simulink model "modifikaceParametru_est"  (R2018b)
settings: Solver=ode4  StartTime=0.0  StopTime=T  FixedStep=1e-3  RelTol=1e-3
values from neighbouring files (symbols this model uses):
  b_1 = params.b_1    [mainSkript_modifikaceParametru.m]    (also in mainSkript_rovniceSystemu.m; mainSkript_overeniRovnic.m; mainSkript_kyvadlaNajednouOdhad.m; mainSkript_simulaceLQG.m)
  b_2 = params.b_2    [mainSkript_modifikaceParametru.m]    (also in mainSkript_rovniceSystemu.m; mainSkript_overeniRovnic.m; mainSkript_kyvadlaNajednouOdhad.m; mainSkript_simulaceLQG.m)
  g = 9.81    [mainSkript_modifikaceParametru.m]    (also in mainSkript_rovniceSystemu.m; mainSkript_overeniRovnic.m; mainSkript_estimaceVozik.m; mainSkript_odhadKyvadlaZvlast.m)
  I_1 = params.I_1    [mainSkript_modifikaceParametru.m]    (also in mainSkript_rovniceSystemu.m; mainSkript_overeniRovnic.m; mainSkript_kyvadlaNajednouOdhad.m; mainSkript_simulaceLQG.m)
  I_2 = params.I_2    [mainSkript_modifikaceParametru.m]    (also in mainSkript_rovniceSystemu.m; mainSkript_overeniRovnic.m; mainSkript_kyvadlaNajednouOdhad.m; mainSkript_simulaceLQG.m)
  L_1 = params.L_1    [mainSkript_modifikaceParametru.m]    (also in mainSkript_rovniceSystemu.m; mainSkript_overeniRovnic.m; odhadovane_parametry.m = 0.228; mainSkript_kyvadlaNajednouOdhad.m)
  l_1 = params.l_1    [mainSkript_modifikaceParametru.m]    (also in mainSkript_rovniceSystemu.m; mainSkript_overeniRovnic.m; odhadovane_parametry.m = 0.134; mainSkript_kyvadlaNajednouOdhad.m)
  l_2 = params.l_2    [mainSkript_modifikaceParametru.m]    (also in mainSkript_rovniceSystemu.m; mainSkript_overeniRovnic.m; odhadovane_parametry.m = 0.112; mainSkript_kyvadlaNajednouOdhad.m)
  m_1 = params.m_1    [mainSkript_modifikaceParametru.m]    (also in mainSkript_rovniceSystemu.m; mainSkript_overeniRovnic.m; mainSkript_kyvadlaNajednouOdhad.m; mainSkript_simulaceLQG.m)
  m_2 = params.m_2    [mainSkript_modifikaceParametru.m]    (also in mainSkript_rovniceSystemu.m; mainSkript_overeniRovnic.m; mainSkript_kyvadlaNajednouOdhad.m; mainSkript_simulaceLQG.m)
  q_0 = [0 pi pi 0 0 0]    [mainSkript_modifikaceParametru.m]    (also in mainSkript_kyvadlaNajednouOdhad.m = cell(1, k); mainSkript_simulaceLQG.m = [0 th1_0 th2_0 0 dth1_0 dth2_0]; mainSkript_LQGexperiment.m = zeros(6,1); mainSkript_LQGexperiment_integral.m = zeros(6,1))

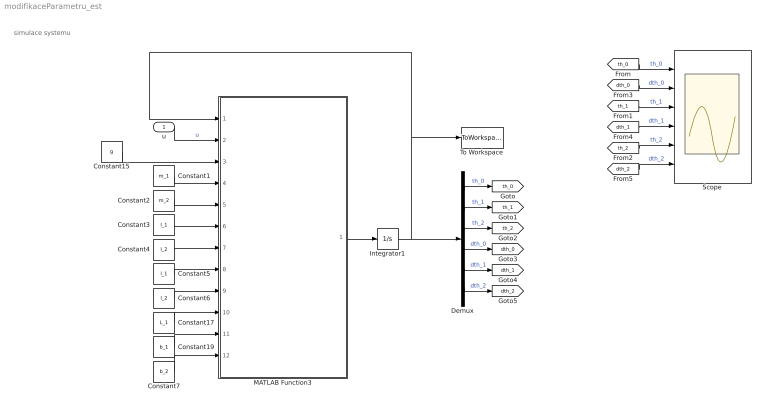
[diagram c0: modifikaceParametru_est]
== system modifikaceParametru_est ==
  note: simulace systemu
  u : Inport
  Constant1 : Constant  Value=m_1
  Constant15 : Constant  Value=g
  Constant17 : Constant  Value=L_1
  Constant19 : Constant  Value=b_1
  Constant2 : Constant  Value=m_2
  Constant3 : Constant  Value=I_1
  Constant4 : Constant  Value=I_2
  Constant5 : Constant  Value=l_1
  Constant6 : Constant  Value=l_2
  Constant7 : Constant  Value=b_2
  Demux : Demux  Outputs=6
  Integrator1 : Integrator  InitialCondition=q_0
  MATLAB Function3 : MATLAB Function  TreatAsAtomicUnit=on
  Scope : Scope  NumInputPorts=6
  To Workspace : ToWorkspace  VariableName=kyvadla  SaveFormat=Structure With Time  SampleTime=-1
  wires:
  Demux/1 -> [th_0]  "th_0"
  Demux/2 -> [th_1]  "th_1"
  Demux/3 -> [th_2]  "th_2"
  Demux/4 -> [dth_0]  "dth_0"
  Demux/5 -> [dth_1]  "dth_1"
  Demux/6 -> [dth_2]  "dth_2"
  [th_0] -> Scope/1  "th_0"
  [th_1] -> Scope/3  "th_1"
  [th_2] -> Scope/5  "th_2"
  [dth_0] -> Scope/2  "dth_0"
  [dth_1] -> Scope/4  "dth_1"
  [dth_2] -> Scope/6  "dth_2"
  u/1 -> MATLAB Function3/2(u)  "u"
  Constant15/1 -> MATLAB Function3/3(g)
  MATLAB Function3/1(dx) -> Integrator1/1
  Integrator1/1 -> Demux/1, To Workspace/1, MATLAB Function3/1(y)
  Constant1/1 -> MATLAB Function3/4(m_1)
  Constant2/1 -> MATLAB Function3/5(m_2)
  Constant3/1 -> MATLAB Function3/6(J_1)
  Constant4/1 -> MATLAB Function3/7(J_2)
  Constant5/1 -> MATLAB Function3/8(l_1)
  Constant6/1 -> MATLAB Function3/9(l_2)
  Constant17/1 -> MATLAB Function3/10(L_1)
  Constant19/1 -> MATLAB Function3/11(b_1)
  Constant7/1 -> MATLAB Function3/12(b_2)

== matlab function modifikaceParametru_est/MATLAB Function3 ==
function dx = PohybovaRceDIP_simplified(y, u, g, m_1, m_2, J_1, J_2, l_1, l_2, L_1, b_1, b_2)
%PohybovaRceDIP_simplified: Zjednodusena pohybova rovnice dvojiteho kyvadla

dx = zeros(6, 1); % definovani sloupcoveho vektoru derivaci stavu 

dx(1) = conj(y(4)); 
dx(2) = conj(y(5)); 
dx(3) = conj(y(6)); 
dx(4) = u; 
dx(5) = conj(y(6))*(((J_2 + l_2^2*m_2)*(b_2 - L_1*l_2*m_2*sin(y(2) - y(3))*y(6)))/(J_1*J_2 + L_1^2*l_2^2*m_2^2 + J_2*L_1^2*m_2 + J_2*l_1^2*m_1 + J_1*l_2^2*m_2 - L_1^2*l_2^2*m_2^2*cos(y(2) - y(3))^2 + l_1^2*l_2^2*m_1*m_2) + (L_1*b_2*l_2*m_2*cos(y(2) - y(3)))/(J_1*J_2 + L_1^2*l_2^2*m_2^2 + J_2*L_1^2*m_2 + J_2*l_1^2*m_1 + J_1*l_2^2*m_2 - L_1^2*l_2^2*m_2^2*cos(y(2) - y(3))^2 + l_1^2*l_2^2*m_1*m_2)) - conj(y(5))*(((b_1 + b_2)*(J_2 + l_2^2*m_2))/(J_1*J_2 + L_1^2*l_2^2*m_2^2 + J_2*L_1^2*m_2 + J_2*l_1^2*m_1 + J_1*l_2^2*m_2 - L_1^2*l_2^2*m_2^2*cos(y(2) - y(3))^2 + l_1^2*l_2^2*m_1*m_2) + (L_1*l_2*m_2*cos(y(2) - y(3))*(b_2 + L_1*l_2*m_2*sin(y(2) - y(3))*y(5)))/(J_1*J_2 + L_1^2*l_2^2*m_2^2 + J_2*L_1^2*m_2 + J_2*l_1^2*m_1 + J_1*l_2^2*m_2 - L_1^2*l_2^2*m_2^2*cos(y(2) - y(3))^2 + l_1^2*l_2^2*m_1*m_2)) - (u*(L_1*l_2^2*m_2^2*cos(y(2)) + J_2*L_1*m_2*cos(y(2)) + J_2*l_1*m_1*cos(y(2)) - L_1*l_2^2*m_2^2*cos(y(2) - y(3))*cos(y(3)) + l_1*l_2^2*m_1*m_2*cos(y(2))))/(J_1*J_2 + L_1^2*l_2^2*m_2^2 + J_2*L_1^2*m_2 + J_2*l_1^2*m_1 + J_1*l_2^2*m_2 - L_1^2*l_2^2*m_2^2*cos(y(2) - y(3))^2 + l_1^2*l_2^2*m_1*m_2) + (g*sin(y(2))*(J_2 + l_2^2*m_2)*(L_1*m_2 + l_1*m_1))/(J_1*J_2 + L_1^2*l_2^2*m_2^2 + J_2*L_1^2*m_2 + J_2*l_1^2*m_1 + J_1*l_2^2*m_2 - L_1^2*l_2^2*m_2^2*cos(y(2) - y(3))^2 + l_1^2*l_2^2*m_1*m_2) - (L_1*g*l_2^2*m_2^2*cos(y(2) - y(3))*sin(y(3)))/(J_1*J_2 + L_1^2*l_2^2*m_2^2 + J_2*L_1^2*m_2 + J_2*l_1^2*m_1 + J_1*l_2^2*m_2 - L_1^2*l_2^2*m_2^2*cos(y(2) - y(3))^2 + l_1^2*l_2^2*m_1*m_2); 
dx(6) = conj(y(5))*(((b_2 + L_1*l_2*m_2*sin(y(2) - y(3))*y(5))*(J_1 + L_1^2*m_2 + l_1^2*m_1))/(J_1*J_2 + L_1^2*l_2^2*m_2^2 + J_2*L_1^2*m_2 + J_2*l_1^2*m_1 + J_1*l_2^2*m_2 - L_1^2*l_2^2*m_2^2*cos(y(2) - y(3))^2 + l_1^2*l_2^2*m_1*m_2) + (L_1*l_2*m_2*cos(y(2) - y(3))*(b_1 + b_2))/(J_1*J_2 + L_1^2*l_2^2*m_2^2 + J_2*L_1^2*m_2 + J_2*l_1^2*m_1 + J_1*l_2^2*m_2 - L_1^2*l_2^2*m_2^2*cos(y(2) - y(3))^2 + l_1^2*l_2^2*m_1*m_2)) - conj(y(6))*((b_2*(J_1 + L_1^2*m_2 + l_1^2*m_1))/(J_1*J_2 + L_1^2*l_2^2*m_2^2 + J_2*L_1^2*m_2 + J_2*l_1^2*m_1 + J_1*l_2^2*m_2 - L_1^2*l_2^2*m_2^2*cos(y(2) - y(3))^2 + l_1^2*l_2^2*m_1*m_2) + (L_1*l_2*m_2*cos(y(2) - y(3))*(b_2 - L_1*l_2*m_2*sin(y(2) - y(3))*y(6)))/(J_1*J_2 + L_1^2*l_2^2*m_2^2 + J_2*L_1^2*m_2 + J_2*l_1^2*m_1 + J_1*l_2^2*m_2 - L_1^2*l_2^2*m_2^2*cos(y(2) - y(3))^2 + l_1^2*l_2^2*m_1*m_2)) - (u*(L_1^2*l_2*m_2^2*cos(y(3)) + J_1*l_2*m_2*cos(y(3)) - L_1^2*l_2*m_2^2*cos(y(2) - y(3))*cos(y(2)) + l_1^2*l_2*m_1*m_2*cos(y(3)) - L_1*l_1*l_2*m_1*m_2*cos(y(2) - y(3))*cos(y(2))))/(J_1*J_2 + L_1^2*l_2^2*m_2^2 + J_2*L_1^2*m_2 + J_2*l_1^2*m_1 + J_1*l_2^2*m_2 - L_1^2*l_2^2*m_2^2*cos(y(2) - y(3))^2 + l_1^2*l_2^2*m_1*m_2) + (g*l_2*m_2*sin(y(3))*(J_1 + L_1^2*m_2 + l_1^2*m_1))/(J_1*J_2 + L_1^2*l_2^2*m_2^2 + J_2*L_1^2*m_2 + J_2*l_1^2*m_1 + J_1*l_2^2*m_2 - L_1^2*l_2^2*m_2^2*cos(y(2) - y(3))^2 + l_1^2*l_2^2*m_1*m_2) - (L_1*g*l_2*m_2*cos(y(2) - y(3))*sin(y(2))*(L_1*m_2 + l_1*m_1))/(J_1*J_2 + L_1^2*l_2^2*m_2^2 + J_2*L_1^2*m_2 + J_2*l_1^2*m_1 + J_1*l_2^2*m_2 - L_1^2*l_2^2*m_2^2*cos(y(2) - y(3))^2 + l_1^2*l_2^2*m_1*m_2);
